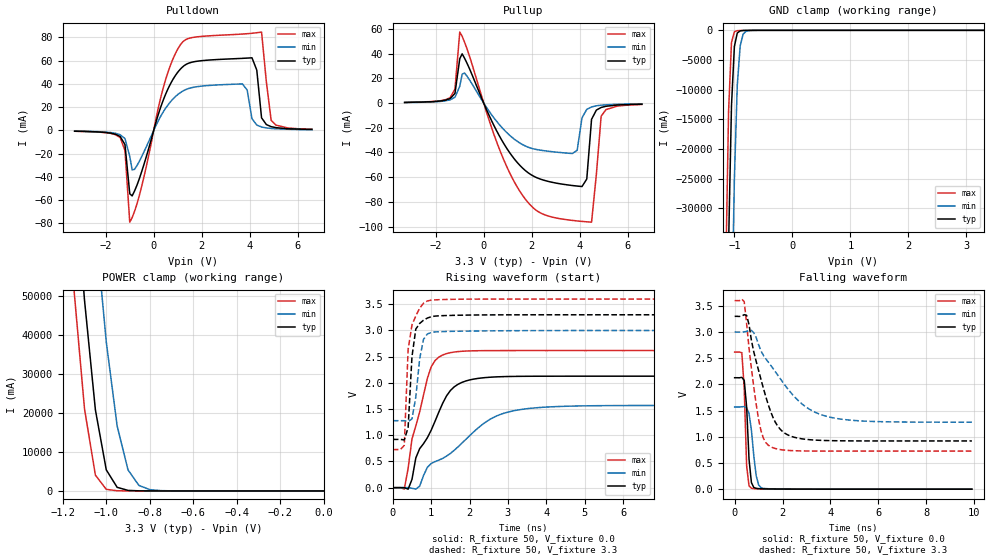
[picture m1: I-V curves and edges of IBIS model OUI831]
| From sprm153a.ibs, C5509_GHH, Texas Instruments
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| Pin_model   OUI831
[Model]   OUI831
 Model_type   3-state
 Polarity   Non-Inverting
 Enable   Active-Low
 Vmeas =  1.5
|Variable   typ   min   max
 C_comp   2.349pF   2.328pF   2.418pF
[Temperature Range]   25   125   -40
[Voltage Range]   3.3   3   3.6
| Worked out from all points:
|   slope of the pulldown table from 0 to 0.495 V, typ, clamps not added: 16 ohm
|   slope of the pullup table from 0 to 0.495 V, typ, clamps not added: 23.8 ohm
|   GND clamp passes 1 mA (typ) near -0.59 V on its own axis
|   POWER clamp passes 1 mA (typ) near -0.70 V on its own axis
|   rising waveform, R_fixture 50, V_fixture 0.0: 20-80 % time 800ps typ, 1.57ns min, 478ps max; typ from 0 V to 2.13 V
|   rising waveform, R_fixture 50, V_fixture 3.3: 20-80 % time 143ps typ, 179ps min, 156ps max; typ from 0.921 V to 3.3 V
|   falling waveform, R_fixture 50, V_fixture 0.0: 20-80 % time 159ps typ, 224ps min, 120ps max; typ from 2.13 V to 0 V
|   falling waveform, R_fixture 50, V_fixture 3.3: 20-80 % time 868ps typ, 1.74ns min, 485ps max; typ from 3.3 V to 0.921 V
[GND Clamp]
|Voltage   I(typ)   I(min)   I(max)
-3.3V     -2.131kA   -2.172kA   -2.112kA
-1.15V    -69.25A    -121A      -41.3A
-1.1V     -36.04A    -83.7A     -13.64A
-1.05V    -12.77A    -50.83A    -2.066A
-1V       -2.725A    -25.08A    -235mA
-950mV    -452.2mA   -9.272A    -58.21mA
-900mV    -87.02mA   -2.634A    -34.85mA
-850mV    -28.65mA   -661.3mA   -25.01mA
-800mV    -15.52mA   -165.1mA   -17.15mA
-600mV    -1.135mA   -2.472mA   -762.4uA
3.3V      201.2pA    2.515nA    171.4pA
[POWER Clamp]
|Voltage   I(typ)   I(min)   I(max)
-3.3V     2.152kA    2.199kA    2.128kA
-1.15V    84.65A     142.8A     52.53A
-1.1V     48.8A      103.8A     20.98A
-1.05V    20.76A     68.2A      4.051A
-1V       5.397A     38.14A     408.9mA
-950mV    921mA      16.63A     39.31mA
-900mV    138.5mA    5.377A     6.91mA
-850mV    22mA       1.408A     3.323mA
-800mV    4.66mA     339.8mA    2.313mA
-750mV    1.713mA    80.91mA    1.624mA
0V        0A         0A         0A
[Pulldown]
|Voltage   I(typ)   I(min)   I(max)
-3.3V     -800uA     -600uA     -800uA
-1.4V     -5.36mA    -3.81mA    -6.26mA
-1.2V     -12.25mA   -7.11mA    -17.31mA
-1V       -54.58mA   -22.44mA   -78.99mA
-800mV    -52.16mA   -33.54mA   -69.68mA
400mV     26.07mA    15.89mA    36.64mA
1.1V      52.31mA    32.25mA    73.11mA
3.7V      61.86mA    39.87mA    82.75mA
4.1V      62.32mA    9.97mA     83.41mA
4.5V      10.72mA    2.83mA     84.43mA
4.9V      3.13mA     1.59mA     8.65mA
6.6V      700uA      600uA      1mA
[Pullup]
|Voltage   I(typ)   I(min)   I(max)
-3.3V     500uA      500uA      600uA
-1.4V     3.68mA     2.67mA     4.45mA
-1.2V     7.89mA     4.73mA     11.41mA
-1V       35.94mA    13.64mA    57.52mA
850mV     -33.18mA   -21.68mA   -46.54mA
2.15V     -59.85mA   -37.37mA   -86.19mA
3.7V      -66.75mA   -40.84mA   -95.02mA
4.1V      -67.58mA   -12.01mA   -95.82mA
4.3V      -61.52mA   -5.05mA    -96.15mA
4.5V      -13.11mA   -3.07mA    -96.45mA
4.9V      -3.53mA    -1.69mA    -10.59mA
6.6V      -900uA     -600uA     -1.1mA
[Ramp]
|Variable   typ   min   max
 dV/dt_r   1.27V/0.800ns   0.94V/1.580ns   1.56V/0.480ns
 dV/dt_f   1.41V/0.860ns   1.04V/1.740ns   1.70V/0.480ns
 R_load =  50
[Rising Waveform]
 R_fixture =   50
 V_fixture =   0.0
 V_fixture_min =  0.0
 V_fixture_max =  0.0
|Time   V(typ)   V(min)   V(max)
0s        10.3nV     2.777uV    10.89nV
300ps     -561.1uV   1.331mV    -27.42mV
500ps     156.2mV    -11.7mV    928.6mV
600ps     566.4mV    -27.88mV   1.177V
900ps     950.9mV    386.8mV    2.082V
1.3ns     1.61V      558.7mV    2.532V
1.9ns     2.036V     919.3mV    2.607V
2.6ns     2.111V     1.332V     2.616V
3.3ns     2.125V     1.487V     2.617V
9.9ns     2.128V     1.569V     2.617V
[Rising Waveform]
 R_fixture =   50
 V_fixture =   3.3
 V_fixture_min =  3
 V_fixture_max =  3.6
|Time   V(typ)   V(min)   V(max)
0s        920.7mV    1.278V     727mV
200ps     921.8mV    1.279V     728mV
300ps     910.6mV    1.278V     808.2mV
400ps     1.149V     1.262V     2.639V
500ps     2.5V       1.312V     3.105V
600ps     3.028V     1.73V      3.277V
700ps     3.134V     2.455V     3.426V
800ps     3.196V     2.83V      3.519V
900ps     3.237V     2.932V     3.563V
9.9ns     3.3V       3V         3.6V
[Falling Waveform]
 R_fixture =   50
 V_fixture =   0.0
 V_fixture_min =  0.0
 V_fixture_max =  0.0
|Time   V(typ)   V(min)   V(max)
0s        2.128V     1.569V     2.617V
300ps     2.135V     1.573V     2.606V
400ps     2.077V     1.577V     1.922V
500ps     1.571V     1.549V     448.1mV
600ps     572.9mV    1.445V     63.48mV
700ps     126mV      1.128V     17.56mV
900ps     15.68mV    253.9mV    7.495mV
1ns       10.34mV    83.17mV    6.011mV
1.2ns     6.44mV     14.73mV    4.091mV
9.9ns     -93.37nV   2.3uV      33.92nV
[Falling Waveform]
 R_fixture =   50
 V_fixture =   3.3
 V_fixture_min =  3
 V_fixture_max =  3.6
|Time   V(typ)   V(min)   V(max)
0s        3.3V       3V         3.6V
400ps     3.332V     3.003V     3.578V
600ps     3.143V     3.028V     2.691V
1ns       2.266V     2.759V     1.332V
1.2ns     1.926V     2.555V     972.8mV
1.5ns     1.484V     2.367V     811.1mV
2.2ns     1.04V      1.925V     741mV
2.9ns     955.5mV    1.595V     729.4mV
3.8ns     928.7mV    1.395V     727mV
9.9ns     920.7mV    1.278V     727mV
